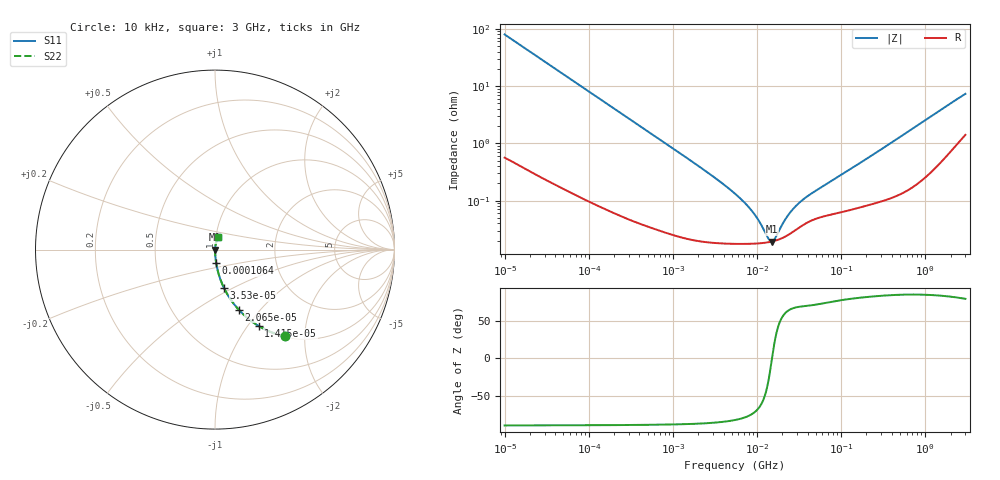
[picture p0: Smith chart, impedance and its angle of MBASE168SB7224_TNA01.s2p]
! MBASE168SB7224_TNA01  S-PARAMETER MODEL  ( Standard Model )
! Model Generated by TAIYO YUDEN Corporation (http://www.ty-top.com)
! Version 1.0
! TAIYO YUDEN Control No. 220601
! Copyright(c) 2012 TAIYO YUDEN CO.,LTD. All Rights Reserved.
! Product Description (link to TY-COMPAS)
! https://ds.yuden.co.jp/TYCOMPAS/or/detail?pn=MBASE168SB7224KTNA01&u=M
! Products Name : Multilayer Ceramic Capacitors
! Characteristics :
!  Capacitance : 0.22 [uF] , Rated Voltage : 16 [V] , TCC : X7R
!  Case Size : 1.6 x 0.8 / 0.063 x 0.031 [mm/inch] , Thickness : 0.8 / 0.031 [mm/inch]
!  (Conditions: Temperature = 25 [degC] , DC Bias Voltage = 0 [V])
! External Node Assignments :
!  1  o---| |---o  2
! GND o---------o GND
! Frequency Range : 10kHz  -  3GHz  [ 401 STEP ]
# MHZ S RI R 50
! Freq[MHz].  S11 Real  S11 Imag  S21 Real  S21 Imag  S12 Real  S12 Imag  S22 Real  S22 Imag
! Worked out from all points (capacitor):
!   401 points, 10 kHz to 3 GHz, reference 50 ohm
!   read as one part in series: C = 200 nF near 10.65 kHz
!   lowest |Z| = 19.3 mohm at 15.02 MHz (marker M1)
!   series resonance near 15.1 MHz, so ESL is about 560 pH
!   S11 on the Smith chart (normalised r, x): 10 kHz: 1.01, -1.59; 14.15 kHz: 1.01, -1.13; 20.65 kHz: 1.01, -0.77; 35.3 kHz: 1.00, -0.45; 106.4 kHz: 1.00, -0.15; 3 GHz: 1.03, +0.14
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0.01  0.3883 -0.4838  0.6117 0.4838  0.6117 0.4838  0.3883 -0.4838
0.014146  0.2426 -0.4248  0.7574 0.4248  0.7574 0.4248  0.2426 -0.4248
0.020651  0.132 -0.3345  0.868 0.3345  0.868 0.3345  0.132 -0.3345
0.035295  0.0507 -0.2148  0.9493 0.2148  0.9493 0.2148  0.0507 -0.2148
0.082683  0.0104 -0.0962  0.9896 0.0962  0.9896 0.0962  0.0104 -0.0962
0.106405  0.00661 -0.0751  0.9934 0.0751  0.9934 0.0751  0.00661 -0.0751
0.683653  0.000443 -0.0119  0.9996 0.0119  0.9996 0.0119  0.000443 -0.0119
2.652321  0.000195 -0.00301  0.9998 0.00301  0.9998 0.00301  0.000195 -0.00301
5.477226  0.000177 -0.00131  0.9998 0.00131  0.9998 0.00131  0.000177 -0.00131
7.048603  0.000176 -0.000919  0.9998 0.000919  0.9998 0.000919  0.000176 -0.000919
8.789267  0.000177 -0.000624  0.9998 0.000624  0.9998 0.000624  0.000177 -0.000624
10.61963  0.00018 -0.000396  0.9998 0.000396  0.9998 0.000396  0.00018 -0.000396
13.66633  0.000188 -0.00011  0.9998 0.00011  0.9998 0.00011  0.000188 -0.00011
15.02209  0.000193 -5.51e-06  0.9998 5.51e-06  0.9998 5.51e-06  0.000193 -5.51e-06
16.51234  0.0002 9.93e-05  0.9998 -9.93e-05  0.9998 -9.93e-05  0.0002 9.93e-05
21.24962  0.000232 0.000383  0.9998 -0.000383  0.9998 -0.000383  0.000232 0.000383
25.67485  0.000274 0.000603  0.9997 -0.000603  0.9997 -0.000603  0.000274 0.000603
33.04079  0.000353 0.000898  0.9996 -0.000898  0.9996 -0.000898  0.000353 0.000898
45.28751  0.000456 0.00128  0.9995 -0.00128  0.9995 -0.00128  0.000456 0.00128
374.4521  0.00117 0.00966  0.9988 -0.00966  0.9988 -0.00966  0.00117 0.00966
1755.269  0.00763 0.0432  0.9924 -0.0432  0.9924 -0.0432  0.00763 0.0432
3000  0.0188 0.0694  0.9812 -0.0694  0.9812 -0.0694  0.0188 0.0694
